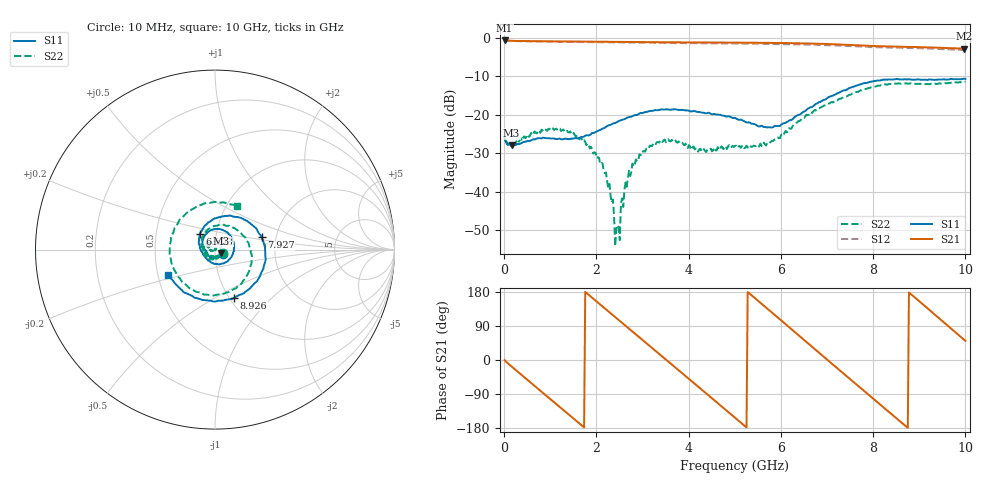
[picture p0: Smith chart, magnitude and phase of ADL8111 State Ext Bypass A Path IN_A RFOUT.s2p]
! Analog Devices Inc.
! Device:  ADL8111
! Description: Bypass Amplifier
! Frequency:  0.00 -  8.00 GHz
! Package:28-Lead Lead Frame Chip Scale Package[LFCSP] 6mm by 6mm
! Conditions:	Vdd = 5.0 V
!		State: External Bypass A
!		Path:  IN_A (Port 1) to RFOUT (Port 2)
!		Idq = 70mA
!		Pin = -10 dBm
!		Temp = +25 C (baseplate temperature)
! Freq(Hz)	S11a(dB)	S11p(deg)	S21a(dB)	S21p(deg)	S12a(dB)	S12p(deg)	S22a(dB)	S22p(deg)
# Hz S  dB  R 50
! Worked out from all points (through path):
!   401 points, 10 MHz to 10 GHz, reference 50 ohm
!   highest |S21| = -0.61 dB at 10 MHz (marker M1); lowest = -2.8 dB at 9.975 GHz (marker M2)
!   group delay of S21, straight-line fit = 286 ps
!   lowest |S11| = -28.0 dB at 159.8 MHz (marker M3), VSWR 1.08, Z = 53.5 - j2.2 ohm
!   |S11| at or under -10 dB: start of sweep to end of sweep
!   |S22| runs from -54.2 to -11.3 dB; largest |S21 - S12| = 0.032
!   S11 on the Smith chart (normalised r, x): 10 MHz: 1.09, -0.05; 6.603 GHz: 0.83, +0.15; 7.927 GHz: 1.68, +0.25; 8.926 GHz: 1.06, -0.62; 10 GHz: 0.57, -0.18
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1e7  -26.12 -26.5  -0.61 -0.6  -0.64 -0.4  -26.17 -22.1
1.5985e8  -27.97 -30.9  -0.69 -17.1  -0.76 -17.0  -28.18 -35.0
9.091e8  -26.08 -126.0  -0.84 -93.8  -0.93 -93.8  -23.90 -147.3
1.683325e9  -25.80 -172.0  -0.92 -172.8  -1.04 -172.8  -26.34 130.0
2.15785e9  -23.49 166.7  -0.94 138.8  -1.09 138.8  -34.57 74.4
2.45755e9  -21.79 148.2  -0.98 108.2  -1.13 108.3  -48.72 -64.0
2.732275e9  -20.53 130.7  -1.01 80.2  -1.17 80.2  -35.97 -161.0
3.35665e9  -18.72 81.4  -1.09 16.4  -1.26 16.5  -27.23 134.9
3.781225e9  -18.71 47.7  -1.10 -26.9  -1.31 -26.8  -26.90 87.7
4.25575e9  -19.32 10.2  -1.13 -75.4  -1.35 -75.4  -28.82 14.3
5.005e9  -20.79 -57.4  -1.18 -152.3  -1.43 -152.2  -28.11 -73.1
5.45455e9  -22.57 -107.4  -1.22 161.4  -1.48 161.6  -28.14 -103.1
5.929075e9  -22.91 -159.3  -1.28 112.4  -1.56 112.6  -25.88 -147.1
6.6034e9  -18.26 133.0  -1.41 42.4  -1.72 42.5  -19.95 130.6
6.678325e9  -17.93 126.0  -1.43 34.6  -1.73 34.7  -19.50 122.5
7.227775e9  -14.39 76.2  -1.64 -22.6  -1.95 -22.4  -16.20 53.5
7.927075e9  -11.41 15.0  -2.01 -94.6  -2.33 -94.5  -12.95 -32.9
8.35165e9  -10.75 -21.9  -2.18 -138.0  -2.49 -137.8  -11.95 -81.1
8.926075e9  -10.81 -68.2  -2.32 162.7  -2.65 162.9  -11.94 -150.0
9.475525e9  -10.79 -109.0  -2.52 105.3  -2.86 105.4  -11.86 134.8
9.975025e9  -10.59 -149.6  -2.77 53.2  -3.14 53.2  -11.34 66.3
1e10  -10.60 -151.5  -2.77 50.5  -3.14 50.7  -11.36 63.6
